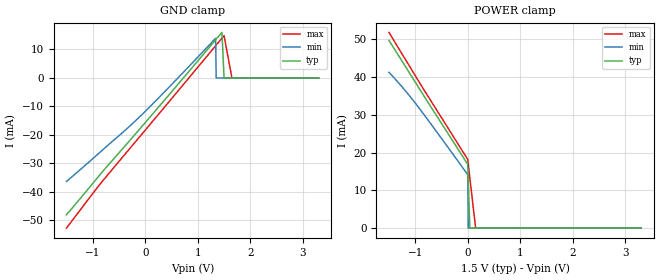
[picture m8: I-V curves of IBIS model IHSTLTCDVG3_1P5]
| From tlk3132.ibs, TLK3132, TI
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|   Model IHSTLTCDVG3_1P5
[Model]   IHSTLTCDVG3_1P5
Model_type   Input
Polarity   Non-Inverting
Vinl =   0.5500V
Vinh =   0.9500V
C_comp   0.7726pF   0.7726pF   0.7726pF
[Temperature Range]   25.0000   0.1250k   -40.0000
[Pullup Reference]   1.5000V   1.3500V   1.6500V
[Pulldown Reference]   0.000V   0.000V   0.000V
[POWER Clamp Reference]   1.5000V   1.3500V   1.6500V
[GND Clamp Reference]   0.000V   0.000V   0.000V
[GND_clamp]
| voltage   I(typ)   I(min)   I(max)
-1.5V     -47.99mA   -36.33mA   -52.68mA
-860mV    -33.9mA    -26.05mA   -37.25mA
-140mV    -18.66mA   -14.21mA   -21.37mA
420mV     -6.613mA   -3.871mA   -9.051mA
1.34V     13.38mA    13.93mA    11.29mA
1.35V     13.82mA    0A         11.74mA
1.46V     16mA       0A         13.95mA
1.5V      0A         0A         14.84mA
1.65V     0A         0A         0A
3.3V      0A         0A         0A
[POWER_clamp]
| voltage   I(typ)   I(min)   I(max)
-1.5V     49.66mA    41.23mA    51.79mA
-1.22V    43.51mA    36.89mA    45.39mA
-960mV    37.76mA    32.39mA    39.44mA
0V        16.87mA    14.12mA    18.17mA
10mV      12.65mA    0A         16.95mA
40mV      0A         0A         13.32mA
150mV     0A         0A         0A
3.3V      0A         0A         0A
